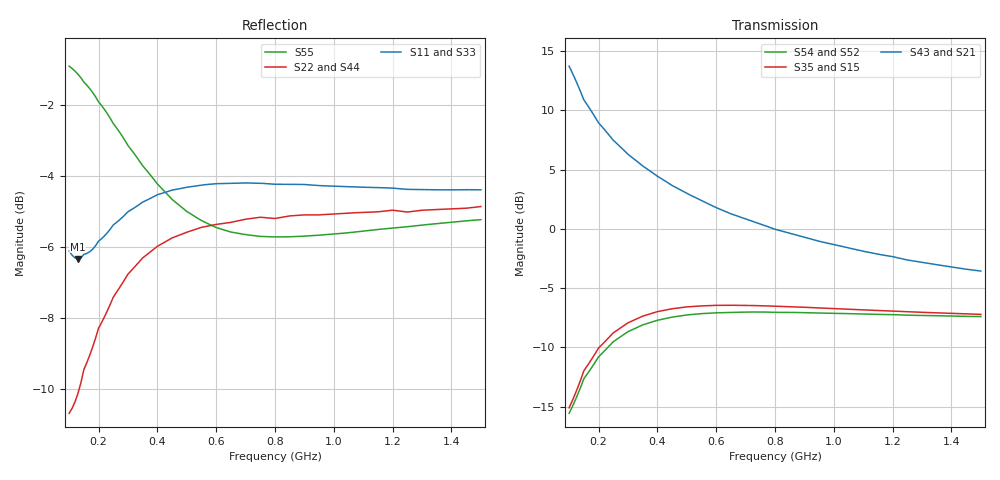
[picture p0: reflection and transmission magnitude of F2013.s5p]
!  POLYFET RF DEVICES
!  F2013
!  S PARAMETERS
!  VDS=28V, IDQ=800mA
! Date: Mon Aug  5 14:20:22 1991
! Bias (V mA) : V1=2.8989000  I1=0.0110650  V2=27.999120  I2=799.60300
!AWR Design Environment (2053) Wed Feb 04 14:47:20 2004
!freq-unit  param-type  data-format  keyword  impedance-ohms
# MHz  S  MA  R  50
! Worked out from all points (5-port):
!   141 points, 100 MHz to 1.5 GHz, reference 50 ohm
!   strongest paths, dB at 100 MHz, 450 MHz, 800 MHz, 1.15 GHz, 1.5 GHz:
!     S43: 13.7, 3.7, 0.0, -2.1, -3.6
!     S21: 13.7, 3.7, 0.0, -2.1, -3.6
!     S35: -15.1, -6.7, -6.5, -6.9, -7.2
!     S15: -15.1, -6.7, -6.5, -6.9, -7.2
!     S54: -15.6, -7.5, -7.0, -7.2, -7.4
!     S52: -15.6, -7.5, -7.0, -7.2, -7.4
!   lowest |S11| = -6.3 dB at 130 MHz (marker M1), VSWR 2.86, Z = 31.5 - j39.5 ohm
!   |S11| at or under -10 dB: nowhere
